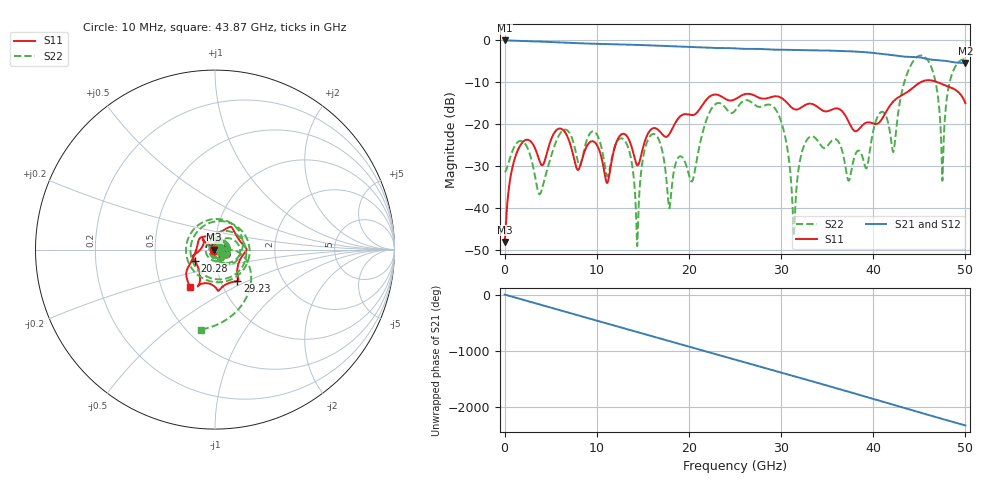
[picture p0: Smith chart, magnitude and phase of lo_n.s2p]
!Keysight Technologies,N5245B,MY57181346,A.12.70.07
!Automatic Fixture Removal (AFR)
!Date: Tuesday, November 06, 2018 3:03:02 PM
!S2P File: Measurements: S11,S21,S12,S22:
# MHz S  RI  R 50
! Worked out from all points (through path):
!   5000 points, 10 MHz to 50 GHz, reference 50 ohm
!   highest |S21| = 0.00 dB at 10 MHz (marker M1); lowest = -5.4 dB at 50 GHz (marker M2)
!   group delay of S21, straight-line fit = 129 ps
!   lowest |S11| = -48.0 dB at 10 MHz (marker M3), VSWR 1.01, Z = 49.6 + j0.0397 ohm
!   |S11| at or under -10 dB: start of sweep to 45.11 GHz; 47.02 GHz to end of sweep
!   |S22| runs from -49.0 to -3.6 dB; largest |S21 - S12| = 1.5e-15
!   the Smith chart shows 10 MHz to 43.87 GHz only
!   S11 on the Smith chart (normalised r, x): 10 MHz: 0.99, +0.00; 20.28 GHz: 0.79, -0.10; 29.23 GHz: 1.20, -0.44; 43.87 GHz: 0.70, -0.31
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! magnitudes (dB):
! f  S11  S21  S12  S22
! 10 MHz  -48.0  0.0  0.0  -31.3
! 2.03 GHz  -24.1  -0.1  -0.1  -24.2
! 3.8 GHz  -28.7  -0.3  -0.3  -36.7
! 6.31 GHz  -21.3  -0.5  -0.5  -21.5
! 8.35 GHz  -28.8  -0.7  -0.7  -28.9
! 12.95 GHz  -22.3  -1.0  -1.0  -23.6
! 14.39 GHz  -29.7  -1.1  -1.1  -49.0
! 15.3 GHz  -23.6  -1.1  -1.1  -25.3
! 16.68 GHz  -21.3  -1.3  -1.3  -23.4
! 17.86 GHz  -22.4  -1.3  -1.3  -40.0
! 20.28 GHz  -17.8  -1.6  -1.6  -33.6
! 22.47 GHz  -13.1  -1.8  -1.8  -16.2
! 25.01 GHz  -14.0  -1.9  -1.9  -16.7
! 29.23 GHz  -13.3  -2.2  -2.2  -15.9
! 31.39 GHz  -16.3  -2.3  -2.3  -46.6
! 33.34 GHz  -15.1  -2.4  -2.4  -22.8
! 37.35 GHz  -19.4  -2.6  -2.6  -33.4
! 41.67 GHz  -16.0  -3.4  -3.4  -20.1
! 43.87 GHz  -12.0  -3.9  -3.9  -6.9
! 46.22 GHz  -9.5  -4.5  -4.5  -5.9
! 47.51 GHz  -10.4  -4.8  -4.8  -33.4
! 50 GHz  -14.9  -5.4  -5.4  -4.5
